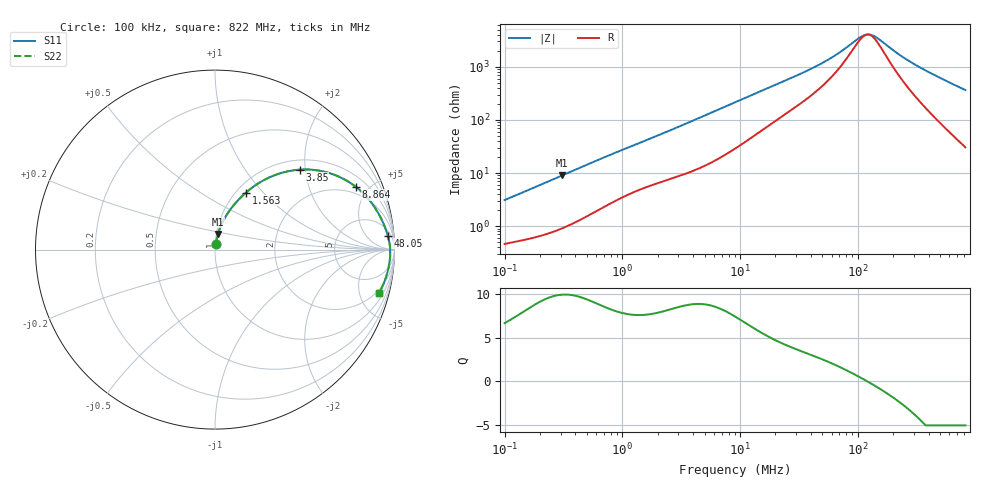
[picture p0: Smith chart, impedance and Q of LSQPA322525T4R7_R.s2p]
! LSQPA322525T4R7_R  S-PARAMETER MODEL  ( General Type )
! Model Generated by TAIYO YUDEN Corporation (http://www.ty-top.com)
! Version 2.0
! TAIYO YUDEN Control No. 100810NF25SB-FKC
! Copyright(c) 2007 TAIYO YUDEN CO.,LTD. All Rights Reserved.
! Product Description (link to TY-COMPAS)
! https://ds.yuden.co.jp/TYCOMPAS/or/detail?pn=LSQPA322525T4R7MR&u=M
! Products Name : Inductors
! Characteristics :
!  Inductance : 4.7 uH , SRF(min) : 70 MHz , DC Resistance(max) : 0.13 Ohm
!  Rated Current : Saturation :1250 mA , Temp Rise : 1010 mA (40 degC)
!  Case Size : 3.2 x 2.5 / 0.126 x 0.098 [mm/inch] , Thickness : 2.5 / 0.098 [mm/inch]
!  (Conditions: Temperature = 25 degC , DC Bias Current/Voltage = 0A / 0V)
! External Node Assignments :
!  1  o---GGG---o  2
! GND o---------o GND
! Frequency Range : 0.1MHz  -  821.96004MHz  [ 402 STEP ]
# MHz S RI R 50
! Freq[MHz].  S11 Real  S11 Imag  S21 Real  S21 Imag  S12 Real  S12 Imag  S22 Real  S22 Imag
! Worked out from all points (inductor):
!   401 points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, 100 kHz to 822 MHz, reference 50 ohm
!   read as one part in series: L = 4.81 uH near 104.6 kHz
!   highest Q = 9.88 at 308.6 kHz (marker M1), where L = 4.65 uH
!   self-resonance near 121.2 MHz
!   S11 on the Smith chart (normalised r, x): 100 kHz: 1.01, +0.06; 1.563 MHz: 1.11, +0.81; 3.85 MHz: 1.21, +1.87; 8.864 MHz: 1.56, +4.17; 48.05 MHz: 9, +21; 822 MHz: 1.61, -7.28
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0.1  0.00555 0.0305  0.9945 -0.0305  0.9945 -0.0305  0.00555 0.0305
0.308572  0.0169 0.0878  0.9831 -0.0878  0.9831 -0.0878  0.0169 0.0878
0.452624  0.0294 0.1246  0.9706 -0.1246  0.9706 -0.1246  0.0294 0.1246
0.889921  0.0811 0.2175  0.9189 -0.2175  0.9189 -0.2175  0.0811 0.2175
1.563254  0.1726 0.3177  0.8274 -0.3177  0.8274 -0.3177  0.1726 0.3177
2.048684  0.2403 0.3683  0.7597 -0.3683  0.7597 -0.3683  0.2403 0.3683
3.850477  0.4721 0.4454  0.5279 -0.4454  0.5279 -0.4454  0.4721 0.4454
5.648013  0.634 0.4274  0.366 -0.4274  0.366 -0.4274  0.634 0.4274
8.864173  0.7861 0.3485  0.2139 -0.3485  0.2139 -0.3485  0.7861 0.3485
9.272834  0.7979 0.339  0.2021 -0.339  0.2021 -0.339  0.7979 0.339
17.03982  0.9028 0.2149  0.0972 -0.2149  0.0972 -0.2149  0.9028 0.2149
41.03579  0.9581 0.0934  0.0419 -0.0934  0.0419 -0.0934  0.9581 0.0934
48.04771  0.963 0.0775  0.037 -0.0775  0.037 -0.0775  0.963 0.0775
64.40289  0.9697 0.0507  0.0303 -0.0507  0.0303 -0.0507  0.9697 0.0507
101.076  0.9751 0.0141  0.0249 -0.0141  0.0249 -0.0141  0.9751 0.0141
115.7099  0.9758 0.00361  0.0242 -0.00361  0.0242 -0.00361  0.9758 0.00361
126.6249  0.9761 -0.00338  0.0239 0.00338  0.0239 0.00338  0.9761 -0.00338
138.5695  0.9763 -0.0104  0.0237 0.0104  0.0237 0.0104  0.9763 -0.0104
185.7378  0.9758 -0.0343  0.0242 0.0343  0.0242 0.0343  0.9758 -0.0343
248.962  0.9735 -0.0611  0.0265 0.0611  0.0265 0.0611  0.9735 -0.0611
341.3129  0.9681 -0.0956  0.0319 0.0956  0.0319 0.0956  0.9681 -0.0956
821.96  0.9128 -0.2434  0.0872 0.2434  0.0872 0.2434  0.9128 -0.2434
